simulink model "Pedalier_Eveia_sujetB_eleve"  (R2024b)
settings: Solver=VariableStepAuto  StartTime=0.0  StopTime=72000  RelTol=1e-3
undefined symbols (not defined in the file): Acid, Lead
libraries: simulink x2, spsBatteryLib x1, spsIdealSwitchLib x1, spsControlledCurrentSourceLib x1, spspowerguiLib x1

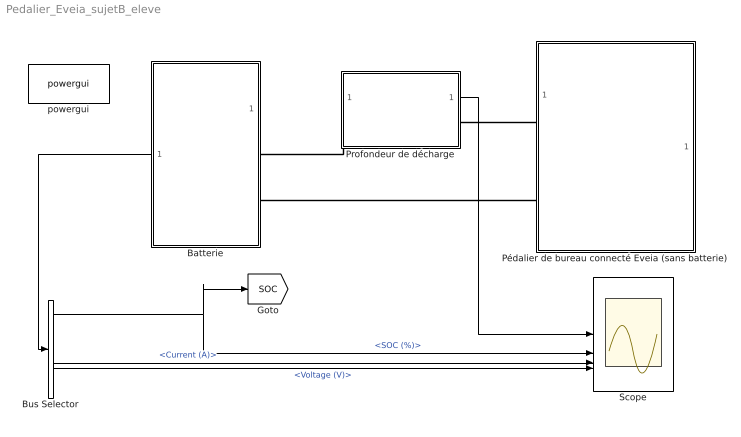
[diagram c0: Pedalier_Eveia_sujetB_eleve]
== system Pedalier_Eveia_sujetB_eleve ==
  Batterie : Subsystem
  Bus Selector : BusSelector  OutputSignals=SOC (%),Current (A),Voltage (V)
  Profondeur de décharge : Subsystem
  Pédalier de bureau connecté Eveia (sans batterie) : Subsystem
  Scope : Scope  NumInputPorts=4
  powergui : spspowerguiLib/powergui  Priority=1  SimulationMode=Continuous  SampleTime=50e-6  frequency=60  Iterations=50  frequencyindice=0  Pbase=100e6  ErrMax=1e-4  UnitsV=kV  UnitsW=MW  buscounter=0  FunctionMessages=off  echomessages=off  EnableUseOfTLC=off  CurrentSourceSwitches=off  DisableSnubberDevices=off  DisableRonSwitches=off  DisableVfSwitches=off  DisplayEquations=off  AutomaticDiscreteSolvers=off  SolverType=Tustin/Backward Euler (TBE)  Interpol=off  ExternalGateDelay=off  methode=off  Ts=100  x0status=blocks  SPID=on  SwTol=0  HookPort=off  NonlinearTolerance=1e-4  nMaxIteration=100  ContinueOnMaxIteration=off  RestoreLinks=warning  ResistiveCurrentMeasurement=off  Frange=[0:2:500]  Ylog=off  Xlog=on  ShowGrid=off  save=off  variable=ZData  structure=0  ZoomFFT=off  StartTime=0.0  cycles=1  DisplayStyle=1  fundamental=60  FreqAxis=off  MaxFrequency=1000  frequencyindicesteady=1  RmsSteady=1  display=off
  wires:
  Bus Selector/1 -> Scope/2, [SOC]  "<SOC (%)>"
  Batterie/1(m) -> Bus Selector/1
  Profondeur de décharge/1(Déchargé ?) -> Scope/1
  Bus Selector/2 -> Scope/3  "<Current (A)>"
  Bus Selector/3 -> Scope/4  "<Voltage (V)>"
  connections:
  Pédalier de bureau connecté Eveia (sans batterie)/LConn1 -- Profondeur de décharge/RConn1
  Profondeur de décharge/LConn1 -- Batterie/LConn1
  Pédalier de bureau connecté Eveia (sans batterie)/LConn2 -- Batterie/LConn2

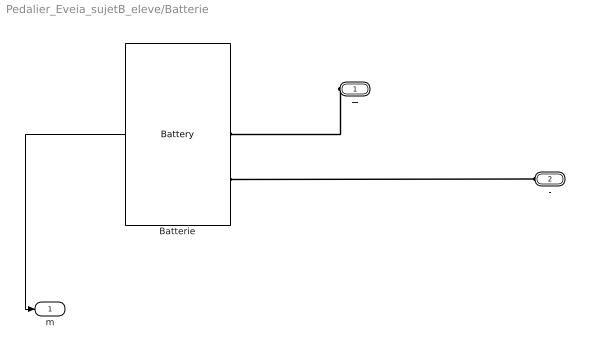
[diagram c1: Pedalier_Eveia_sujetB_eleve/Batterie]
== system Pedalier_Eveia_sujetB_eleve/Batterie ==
  Batterie : spsBatteryLib/Battery  BatType=Lead-Acid  NomV=0  NomQ=0  SOC=100  Batt_Tr=1  PresetModel=on  MaxQ=0  MinV=0  FullV=0  Dis_rate=0  R=NaN  Normal_OP=0  expZone="[0  0]"
  + : PMIOPort  Side=Left
  - : PMIOPort  Port=2  Side=Left
  m : Outport
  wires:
  Batterie/1 -> m/1
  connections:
  -/RConn1 -- Batterie/LConn2
  +/RConn1 -- Batterie/LConn1

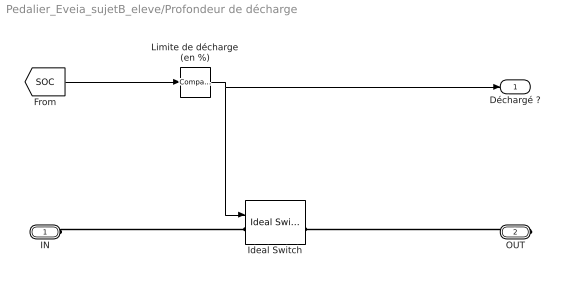
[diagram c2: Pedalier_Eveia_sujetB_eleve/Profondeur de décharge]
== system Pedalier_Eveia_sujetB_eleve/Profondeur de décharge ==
  Ideal Switch : spsIdealSwitchLib/Ideal Switch  Ron=0.001  Lon=0  IC=1  Rs=1e5  Cs=inf  Measurements=on
  Limite de décharge (en %) : simulink/Logic and Bit Operations/Compare To Constant  relop=>=  const=20  OutDataTypeStr=uint8
  IN : PMIOPort  Side=Left
  OUT : PMIOPort  Port=2  Side=Right
  Déchargé ? : Outport
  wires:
  Limite de décharge (en %)/1 -> Déchargé ?/1, Ideal Switch/1
  [SOC] -> Limite de décharge (en %)/1
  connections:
  IN/RConn1 -- Ideal Switch/LConn1
  OUT/RConn1 -- Ideal Switch/RConn1

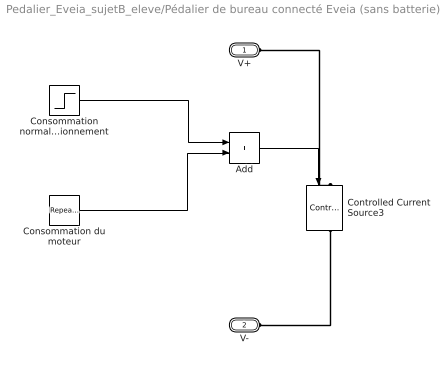
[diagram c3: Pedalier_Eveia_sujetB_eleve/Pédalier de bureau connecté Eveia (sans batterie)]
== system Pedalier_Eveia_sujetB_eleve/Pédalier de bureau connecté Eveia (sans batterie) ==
  Add : Sum
  Consommation du moteur : simulink/Sources/Repeating Sequence Stair  OutValues=[0 0 0 0 0 0 0 0 0 0 0 0 0 0 0 0 0 0 0 0 0 0 0 0 0 0 0 0 0 0 0 0 0 0 0 0 0 0 0 0 0 0 0 0 0 0 0 0 0 0 0 0 0 0 0 0 0 0 0 0.2].'  tsamp=5  OutMin=[]  OutMax=[]  OutDataTypeStr=double  OutputDataTypeScalingMode=double  OutDataType=fixdt(0,8)  ConRadixGroup=Best Precision: Vector-wise  OutScaling=2^-12
  Consommation normale de fonctionnement : Step  After=0.2  SampleTime=0
  Controlled Current Source3 : spsControlledCurrentSourceLib/Controlled Current Source  Initialize=on  Source_Type=DC  Amplitude=0  Phase=0  Frequency=0  Measurements=None
  V+ : PMIOPort  Side=Left
  V- : PMIOPort  Port=2  Side=Left
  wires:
  Add/1 -> Controlled Current Source3/1
  Consommation normale de fonctionnement/1 -> Add/1
  Consommation du moteur/1 -> Add/2
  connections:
  Controlled Current Source3/RConn1 -- V-/RConn1
  V+/RConn1 -- Controlled Current Source3/LConn1
